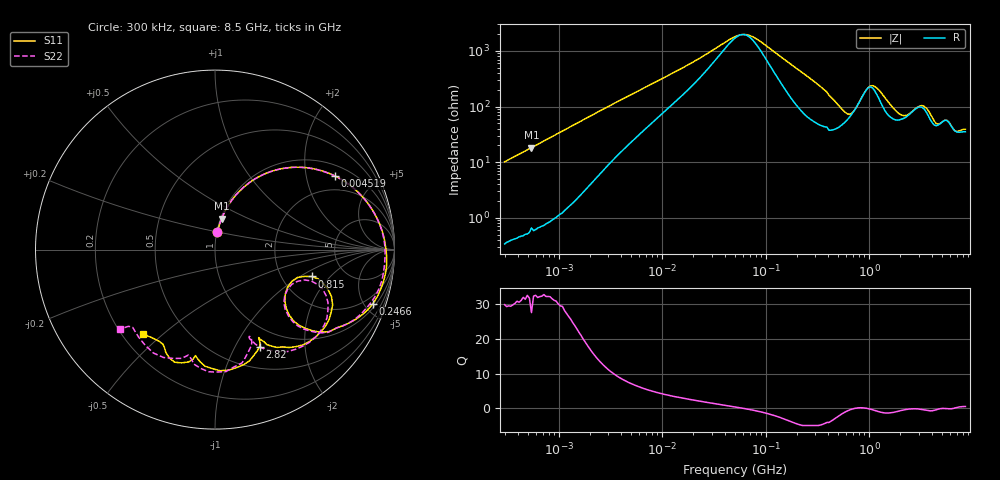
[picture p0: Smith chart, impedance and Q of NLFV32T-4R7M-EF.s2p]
! S-parameter Generated by TDK Corporation
! Copyright(C) 2015 TDK Corporation.
! All Rights Reserved.
! TDK P/N: NLFV32T-4R7M-EF (Inductors)
! Property: L=4.7uH at 7.96MHz
! Size(LxWxT): 3.2x2.5x2.2mm, 0.126x0.098x0.087inches
! Model Type: s2p (Touchstone File Format Version 1.0)
! Frequency: DC=Yes Start=0.3MHz Stop=8500MHz 225points Log-sweep
! Note:
! Model Generated on Jun. 23, 2015
! Hash(MD5):
! Port Assignments:
!  1 ---@@@--- 2
! Applicable Conditions:
!  Temperature = 25 degC
!  DC Bias Current = 0 A
!  Small Signal Operation
! Terms and conditions regarding TDK Simulation Models
! (1)This simulation model is being provided solely for informational purposes. Please refer to the specifications of the products in terms of detailed characteristics of such products.
! (2)In no event shall TDK Corporation of any of its subsidiaries be liable for any loss or damage arising, directly or indirectly,
!  From any information contained in this simulation model, including, but not limited to loss or damages arising from any inaccuracies, omissions or errors in connection with such information.
! (3)Any and all copyrights on this simulation model are owned by TDK Corporation.
!  Duplication or redistribution of this simulation model without prior written permission from TDK Corporation is prohibited.
! (4)This simulation model is subject to any modification or change without any prior notice.
! (5)Neither TDK Corporation nor any of its subsidiaries shall make any warranty, express or implied,
!  Including but not limited to the correctness, implied warranties of merchantability and fitness for a particular purpose with respect to this simulation models.
! (6)The use of this simulation model shall be deemed to have consented to the terms and conditions hereof.
# MHz S MA R 50
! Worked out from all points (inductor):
!   224 points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, 300 kHz to 8.5 GHz, reference 50 ohm
!   read as one part in series: L = 5.35 uH near 314.1 kHz
!   highest Q = 32.4 at 545.3 kHz (marker M1), where L = 5.29 uH
!   self-resonance near 59.35 MHz
!   S11 on the Smith chart (normalised r, x): 300 kHz: 1.01, +0.20; 4.519 MHz: 1.38, +2.95; 246.6 MHz: 1.28, -5.67; 815 MHz: 2.93, -1.28; 2.82 GHz: 0.75, -1.26; 8.5 GHz: 0.28, -0.43
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0.3  0.09875 82.5  0.9894 -5.7  0.9939 -6.0  0.09818 82.6
0.5453461  0.1764 77.6  0.9773 -10.2  0.9792 -10.4  0.1755 77.9
1.72111  0.4871 58.0  0.8498 -29.1  0.8511 -29.5  0.4875 58.0
4.519427  0.7846 31.5  0.529 -51.1  0.5295 -51.5  0.7849 31.4
9.430415  0.8913 16.6  0.2967 -60.5  0.2969 -60.8  0.8914 16.5
51.67171  0.9529 -0.1  0.05179 -17.1  0.05183 -17.4  0.9476 -0.4
78.15234  0.9582 -3.2  0.05537 30.6  0.0554 30.2  0.9483 -3.6
246.6485  0.9289 -19.1  0.2518 60.0  0.2519 59.6  0.9127 -19.7
283.1228  0.9077 -22.5  0.2973 56.7  0.2975 56.4  0.8933 -23.1
448.3627  0.7353 -38.5  0.5105 35.5  0.511 35.0  0.7273 -39.3
590.7752  0.5148 -39.5  0.5939 11.4  0.5941 11.1  0.5135 -40.4
678.1388  0.4556 -27.2  0.5642 -3.0  0.5644 -3.3  0.461 -28.8
815.0429  0.5601 -15.5  0.4346 -17.2  0.4352 -17.4  0.5625 -18.0
1073.923  0.7365 -28.7  0.2876 -2.1  0.2867 -2.1  0.7308 -31.4
1551.304  0.6841 -52.9  0.4575 6.1  0.4579 5.3  0.6771 -57.1
2044.041  0.5645 -63.0  0.5322 -14.2  0.5327 -14.3  0.5499 -67.8
2819.992  0.595 -65.3  0.4358 -34.7  0.4355 -35.5  0.571 -69.2
3890.506  0.6754 -87.6  0.429 -31.4  0.4298 -32.0  0.6814 -93.1
4895.91  0.6 -100.4  0.4692 -52.2  0.4706 -53.4  0.606 -104.2
6161.135  0.6663 -109.7  0.4118 -61.3  0.4075 -61.5  0.6705 -120.8
7404.957  0.602 -118.7  0.4217 -78.4  0.4226 -79.1  0.6309 -136.5
8500  0.6182 -130.5  0.3465 -94.6  0.3455 -93.9  0.6904 -140.0
